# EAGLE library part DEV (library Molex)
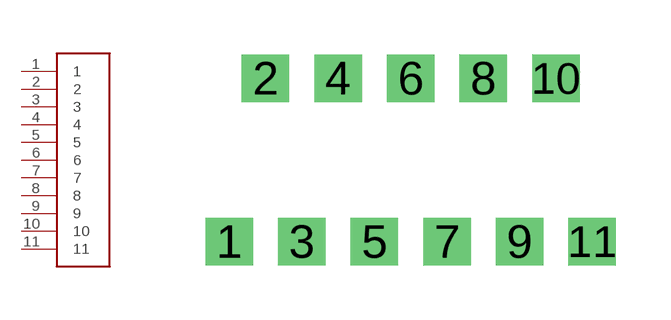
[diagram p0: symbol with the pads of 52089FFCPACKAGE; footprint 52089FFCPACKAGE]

Designator prefix MOLEX_MOTOR

## DEV  [52089FFCPACKAGE]
1  1
2  2
3  3
4  4
5  5
6  6
7  7
8  8
9  9
10  10
11  11

## Footprint 52089FFCPACKAGE (pad centres in mm)
drill 0.8 square: 1 0,0; 2 1,4.5; 3 2,0; 4 3,4.5; 5 4,0; 6 5,4.5; 7 6,0; 8 7,4.5; 9 8,0; 10 9,4.5; 11 10,0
